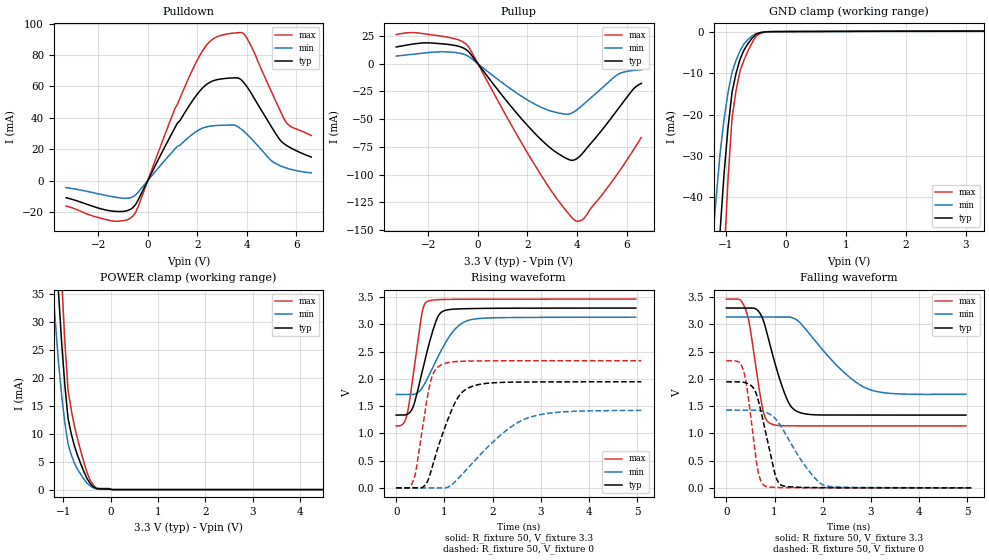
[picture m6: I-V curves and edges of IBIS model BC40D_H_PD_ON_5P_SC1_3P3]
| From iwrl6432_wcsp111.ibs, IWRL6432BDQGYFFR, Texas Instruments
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|   Model Cell BC40D_H_PD_ON_5P_SC1_3P3
|BC40D_H_PD_ON_5P_SC1_3P3
[Model]   BC40D_H_PD_ON_5P_SC1_3P3
Model_type   I/O
Polarity   Non-Inverting
Enable   Active-Low
Vinl =  0.8V
Vinh =  2V
Cref =  15pF
Rref =  100.0000M
Vref =  0V
Vmeas =  1.65
C_comp   2.157014p   1.964007p   2.198404p
|[Input load] weak_pd_on
|[Output drive] slow
|[supplytol] 5
|[temp] ind
[Model Spec]
Vinl   0.8V   0.8V   0.8V
Vinh   2V   2V   2V
[Temperature Range]   25   125   -40
[Voltage Range]   3.3   3.135   3.465
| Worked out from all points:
|   slope of the pulldown table from 0 to 0.495 V, typ, clamps not added: 31.8 ohm
|   slope of the pullup table from 0 to 0.495 V, typ, clamps not added: 33.8 ohm
|   GND clamp passes 1 mA (typ) near -0.52 V on its own axis
|   POWER clamp passes 1 mA (typ) near -0.42 V on its own axis
|   rising waveform, R_fixture 50, V_fixture 3.3: 20-80 % time 338ps typ, 517ps min, 220ps max; typ from 1.33 V to 3.3 V
|   rising waveform, R_fixture 50, V_fixture 0: 20-80 % time 469ps typ, 1.01ns min, 253ps max; typ from 0 V to 1.95 V
|   falling waveform, R_fixture 50, V_fixture 3.3: 20-80 % time 388ps typ, 896ps min, 241ps max; typ from 3.3 V to 1.33 V
|   falling waveform, R_fixture 50, V_fixture 0: 20-80 % time 295ps typ, 612ps min, 205ps max; typ from 1.95 V to 0 V
| Nom Voltages:
|   VDD=1.1, VDDS=3.3, VDDS18=1.8, ESD_BIASFET=0, VSS=0, VSSS=0
| Min Voltages:
|   VDD=1.045, VDDS=3.135, VDDS18=1.71, ESD_BIASFET=0, VSS=0, VSSS=0
| Max Voltages:
|   VDD=1.16, VDDS=3.465, VDDS18=1.89, ESD_BIASFET=0, VSS=0, VSSS=0
[POWER_clamp]
|   voltage   I(typ)   I(min)   I(max)
-3.3V     446.9mA    437.1mA    604mA
-1.233V   56.59mA    37.52mA    80.37mA
-1.167V   45.68mA    29.91mA    65.17mA
-1.1V     35.14mA    22.67mA    50.36mA
-1.033V   26.13mA    16.78mA    37.31mA
-966.7mV  18.67mA    11.95mA    26.46mA
-900mV    12.76mA    8.173mA    17.82mA
-833.3mV  10.07mA    6.293mA    14.34mA
-566.7mV  3.276mA    1.91mA     4.968mA
-366.7mV  519.9uA    314uA      774.5uA
33.33mV   0A         0A         0A
6.6V      0A         0A         0A
[Pulldown]
|   voltage   I(typ)   I(min)   I(max)
-3.3V     -10.93mA   -4.474mA   -16.27mA
-1.4V     -19.53mA   -10.38mA   -25.83mA
-600mV    -17.23mA   -10.34mA   -22.61mA
1.2V      36.72mA    21.93mA    48.76mA
1.9V      53.02mA    30.66mA    73.76mA
2.4V      61.61mA    34.34mA    86.89mA
3V        64.86mA    35.24mA    92.76mA
3.6V      65.51mA    34.65mA    94.24mA
3.9V      62.01mA    31.1mA     93.16mA
5V        34.1mA     12.57mA    56.42mA
5.6V      22.42mA    7.958mA    36.79mA
6.6V      14.97mA    4.886mA    28.74mA
[Pullup]
|   voltage   I(typ)   I(min)   I(max)
-3.3V     15.12mA    6.907mA    26.36mA
-1.9V     18.73mA    10.27mA    26.12mA
-900mV    16.4mA     10.09mA    22.38mA
-400mV    11.39mA    6.888mA    15.9mA
1.3V      -37.44mA   -22.28mA   -53.31mA
2.5V      -67.31mA   -38.74mA   -98.62mA
3.5V      -84.52mA   -45.4mA    -130.8mA
4V        -85.48mA   -41.54mA   -142.1mA
4.3V      -78.82mA   -35.86mA   -139.1mA
5.6V      -42.54mA   -10.35mA   -100.5mA
6.3V      -22.29mA   -5.95mA    -77mA
6.6V      -17.71mA   -5.359mA   -66.44mA
[GND_clamp]
|   voltage   I(typ)   I(min)   I(max)
-3.3V     -787.2mA   -627.7mA   -1.235A
-1.233V   -85.66mA   -52.14mA   -138.8mA
-1.167V   -66.47mA   -40.37mA   -107.7mA
-1.1V     -48.25mA   -29.37mA   -77.98mA
-1.033V   -34.28mA   -21.19mA   -54.56mA
-966.7mV  -23.07mA   -14.67mA   -35.51mA
-900mV    -14.62mA   -9.792mA   -20.84mA
-833.3mV  -10.07mA   -6.939mA   -14.17mA
-700mV    -4.435mA   -2.94mA    -6.836mA
-500mV    -641.2uA   -454.9uA   -1.12mA
-300mV    -31.62uA   -32.88uA   -44.11uA
3.3V      108.6uA    60.68uA    188uA
[Ramp]
| variable   typ   min   max
dV/dt_f  1.1800167/0.38879191n 0.85627032/0.90202357n   1.397609/0.24104105n
dV/dt_r   1.173121/0.47024854n 0.86169199/1.0194137n  1.4054523/0.25425147n
R_load = 50
[Rising Waveform]
R_fixture = 50
V_fixture = 3.3
V_fixture_min = 3.135
V_fixture_max = 3.465
|   time   V(typ)   V(min)   V(max)
0s        1.335V     1.713V     1.137V
142.6ps   1.335V     1.713V     1.174V
221.5ps   1.347V     1.713V     1.333V
358.2ps   1.503V     1.714V     2.101V
530.2ps   2.098V     1.822V     3.182V
644.3ps   2.513V     2V         3.418V
917.7ps   3.206V     2.493V     3.454V
1.205ns   3.279V     2.896V     3.459V
1.506ns   3.288V     3.074V     3.46V
4.974ns   3.298V     3.131V     3.462V
[Rising Waveform]
R_fixture = 50
V_fixture = 0
V_fixture_min = 0
V_fixture_max = 0
|   time   V(typ)   V(min)   V(max)
0s        0V         0V         0V
263.8ps   0V         0V         0V
361.7ps   0V         0V         145.6mV
579.9ps   30.57mV    0V         1.306V
709.1ps   267.2mV    0V         1.934V
934.7ps   919.6mV    0V         2.257V
1.283ns   1.66V      167.6mV    2.319V
1.636ns   1.879V     508.1mV    2.328V
2.802ns   1.943V     1.303V     2.332V
5.089ns   1.946V     1.421V     2.333V
[Falling Waveform]
R_fixture = 50
V_fixture = 3.3
V_fixture_min = 3.135
V_fixture_max = 3.465
|   time   V(typ)   V(min)   V(max)
0s        3.298V     3.133V     3.461V
275.8ps   3.298V     3.133V     3.454V
414.2ps   3.298V     3.133V     3.24V
753.8ps   3.104V     3.133V     1.452V
907.6ps   2.62V      3.133V     1.183V
1.258ns   1.627V     3.133V     1.138V
1.515ns   1.384V     3.04V      1.137V
2.33ns    1.336V     2.213V     1.136V
2.908ns   1.335V     1.826V     1.136V
4.974ns   1.334V     1.716V     1.136V
[Falling Waveform]
R_fixture = 50
V_fixture = 0
V_fixture_min = 0
V_fixture_max = 0
|   time   V(typ)   V(min)   V(max)
0s        1.945V     1.426V     2.332V
352.9ps   1.938V     1.426V     2.156V
435.9ps   1.916V     1.426V     1.787V
653.6ps   1.634V     1.423V     327.2mV
798.8ps   1.089V     1.391V     35.32mV
1.023ns   216.2mV    1.265V     7.378mV
1.176ns   37.04mV    1.069V     3.545mV
1.667ns   7.041mV    365.6mV    0V
2.037ns   3.675mV    44.94mV    0V
5.089ns   0V         0V         0V
